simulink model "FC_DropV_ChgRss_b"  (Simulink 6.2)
settings: Solver=ode4  SolverMode=SingleTasking  StartTime=0.0  StopTime=1  FixedStep=1e-5  MaxStep=1e-4  RelTol=1e-3

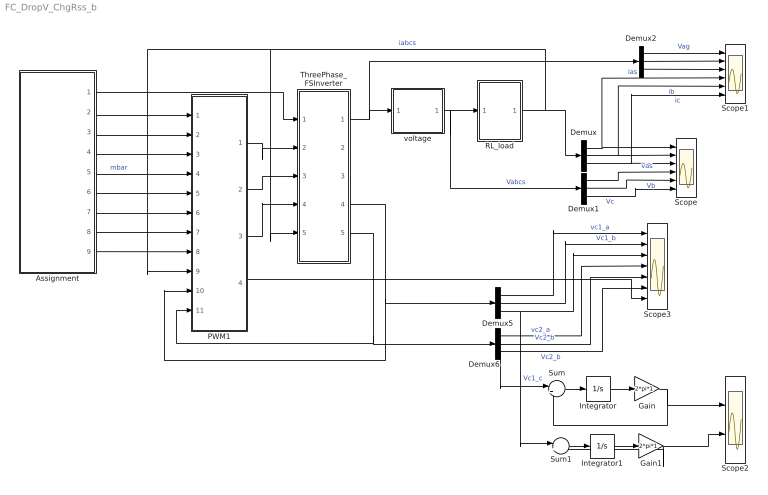
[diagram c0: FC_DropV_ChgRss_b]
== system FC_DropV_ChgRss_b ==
  Assignment : Subsystem  mask{V1Ratio=1, V2Ratio=2, V3Ratio=4, Vdc=50, fe=60, mbar=1.14}
      mask init:
      | Vc1 = Vdc*V1Ratio/V3Ratio;
      | Vc2 = Vdc*V2Ratio/V3Ratio;
  Demux{,1..2,5..6} (5 alike) : Demux  Outputs=3
  Gain : Gain  Gain=2*pi*1
  Gain1 : Gain  Gain=2*pi*1
  Integrator : Integrator
  Integrator1 : Integrator
  PWM1 : Subsystem  AncestorBlock=IMLibrary/PWM1  mask{JustVal=Left Justified, fsw=5e3, F3ndH=on}
      mask prompts: JustVal "Justification"; F3ndH "with the 3nd harmonic injection"
  RL_load : Subsystem  AncestorBlock=IMLibrary/RL_load  mask{Imp=5.37, pf=0.8}
      mask prompts: Imp "Impedance  magnitude"
      mask init:
      | R = pf*Imp;
      | X = sqrt(Imp^2-R^2);
      | L = X/(2*pi*60)
  Scope : Scope  NumInputPorts=6
  Scope1 : Scope  NumInputPorts=6
  Scope2 : Scope  NumInputPorts=2
  Scope3 : Scope  NumInputPorts=7
  Sum : Sum  Inputs=|+-
  Sum1 : Sum  Inputs=|+-
  ThreePhase_FSInverter : Subsystem  AncestorBlock=IMLibrary/ThreePhase_FSInverter  mask{C1=3300e-6, C2=3300e-6, Vc1_a=12.5, Vc2_a=25, Vc1_b=12.5, Vc2_b=25, Vc1_c=12.5, Vc2_c=25}
      mask prompts: Vc1_a "Vc1_a(capacitors initial values)"; Vc2_a "Vc2_a(capacitors initial values)"
  voltage : Subsystem  AncestorBlock=IMLibrary/voltage
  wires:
  Assignment/2(t) -> PWM1/1(t)
  Assignment/4(NLevel) -> PWM1/3(NLevel)
  Assignment/5(mbar) -> PWM1/4(mbar)  "mbar"
  Assignment/6(Vc1_com) -> PWM1/5(V1_com)
  Assignment/7(Vc2_com) -> PWM1/6(V2_com)
  Assignment/8(RSSTable) -> PWM1/7(RSSTable)
  Assignment/9(RSSTable1) -> PWM1/8(RSSTable1)
  Assignment/1(Vdc) -> ThreePhase_FSInverter/1(Vdc)
  ThreePhase_FSInverter/5(Vc2) -> Demux6/1, PWM1/11(V2)
  ThreePhase_FSInverter/4(Vc1) -> Demux5/1, PWM1/10(V1)
  Assignment/3(Theata_c) -> PWM1/2(Theata_c)
  ThreePhase_FSInverter/1(Vabcg) -> Demux2/1, voltage/1(Vabcg)
  PWM1/1(T1) -> ThreePhase_FSInverter/2(T1)
  PWM1/2(T2) -> ThreePhase_FSInverter/3(T2)
  PWM1/3(T3) -> ThreePhase_FSInverter/4(T3)
  voltage/1(Vabcs) -> Demux1/1, RL_load/1(Vabcs)  "Vabcs"
  RL_load/1(iabcs) -> Demux/1, ThreePhase_FSInverter/5(iabcs), PWM1/9(is)  "iabcs"
  Demux/1 -> Scope/1, Scope1/4  "ias"
  Demux/2 -> Scope/2, Scope1/5  "ib"
  Demux/3 -> Scope/3, Scope1/6  "ic"
  Demux2/1 -> Scope1/1  "Vag"
  Demux2/2 -> Scope1/2
  Demux2/3 -> Scope1/3
  PWM1/4(FdeltVPN) -> Scope3/7
  Demux5/3 -> Scope3/3, Sum1/1  "Vc1_c"
  Demux6/3 -> Scope3/6, Sum/1  "Vc2_b"
  Demux5/1 -> Scope3/1  "vc1_a"
  Demux5/2 -> Scope3/2  "Vc1_b"
  Demux6/1 -> Scope3/4  "vc2_a"
  Demux6/2 -> Scope3/5  "Vc2_b"
  Sum/1 -> Integrator/1
  Integrator/1 -> Gain/1
  Gain/1 -> Sum/2, Scope2/1
  Sum1/1 -> Integrator1/1
  Integrator1/1 -> Gain1/1
  Gain1/1 -> Sum1/2, Scope2/2
  Demux1/1 -> Scope/4  "vas"
  Demux1/2 -> Scope/5  "Vb"
  Demux1/3 -> Scope/6  "Vc"

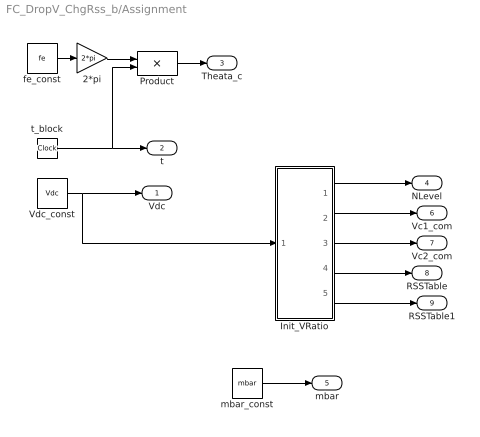
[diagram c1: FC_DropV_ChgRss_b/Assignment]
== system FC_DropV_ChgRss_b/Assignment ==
  2*pi : Gain  Gain=2*pi
  Init_VRatio : Subsystem  AncestorBlock=IMLibrary/Init_VRatio  mask{V1Ratio=V1Ratio, V2Ratio=V2Ratio, V3Ratio=V3Ratio}
  Product : Product
  Vdc_const : Constant  Value=Vdc
  fe_const : Constant  Value=fe
  mbar_const : Constant  Value=mbar
  t_block : Clock
  Vdc : Outport
  t : Outport  Port=2
  Theata_c : Outport  Port=3
  NLevel : Outport  Port=4
  mbar : Outport  Port=5
  Vc1_com : Outport  Port=6
  Vc2_com : Outport  Port=7
  RSSTable : Outport  Port=8
  RSSTable1 : Outport  Port=9
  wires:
  t_block/1 -> t/1, Product/2
  Vdc_const/1 -> Vdc/1, Init_VRatio/1(Vdc)
  Init_VRatio/5(RSSTable1) -> RSSTable1/1
  mbar_const/1 -> mbar/1
  Product/1 -> Theata_c/1
  Init_VRatio/4(RSSTable) -> RSSTable/1
  Init_VRatio/3(Vc2_c) -> Vc2_com/1
  Init_VRatio/2(Vc1_c) -> Vc1_com/1
  Init_VRatio/1(NLevel) -> NLevel/1
  fe_const/1 -> 2*pi/1
  2*pi/1 -> Product/1

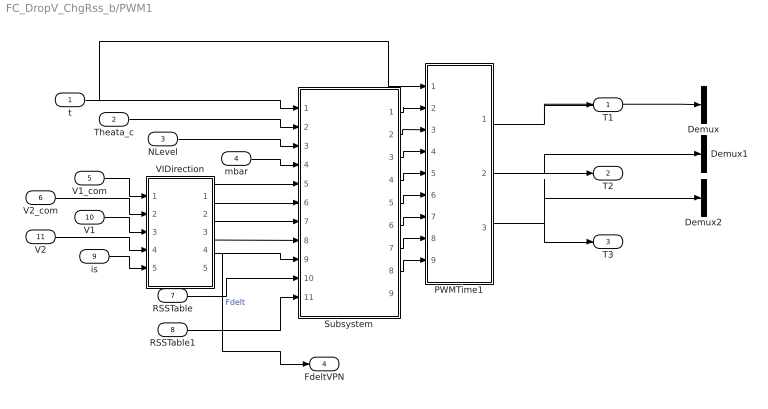
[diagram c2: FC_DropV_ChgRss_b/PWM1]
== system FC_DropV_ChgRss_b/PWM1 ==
  t : Inport  Port=1  LatchInput=off
  Theata_c : Inport  Port=2  LatchInput=off
  NLevel : Inport  Port=3  LatchInput=off
  mbar : Inport  Port=4  LatchInput=off
  V1_com : Inport  Port=5  LatchInput=off
  V2_com : Inport  Port=6  LatchInput=off
  RSSTable : Inport  Port=7  LatchInput=off
  RSSTable1 : Inport  Port=8  LatchInput=off
  is : Inport  Port=9  LatchInput=off
  V1 : Inport  Port=10  LatchInput=off
  V2 : Inport  Port=11  LatchInput=off
  Demux : Demux  Outputs=3
  Demux1 : Demux  Outputs=3
  Demux2 : Demux  Outputs=3
  PWMTime1 : Subsystem
  Subsystem : Subsystem
  VIDirection : Subsystem
  T1 : Outport
  T2 : Outport  Port=2
  T3 : Outport  Port=3
  FdeltVPN : Outport  Port=4
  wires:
  RSSTable1/1 -> Subsystem/11(RSSTable1)
  RSSTable/1 -> Subsystem/10(RSSTable)
  mbar/1 -> Subsystem/4(mbar)
  Theata_c/1 -> Subsystem/2(theta)
  VIDirection/1(FV1) -> Subsystem/5(Fv1)
  VIDirection/2(FV2) -> Subsystem/6(Fv2)
  VIDirection/3(Fis) -> Subsystem/7(Fis)
  V1_com/1 -> VIDirection/1(V1_c)
  V2_com/1 -> VIDirection/2(V2_c)
  is/1 -> VIDirection/5(is)
  VIDirection/4(FDeltVP) -> Subsystem/8(Fdeltp)
  V1/1 -> VIDirection/3(V1)
  V2/1 -> VIDirection/4(V2)
  t/1 -> PWMTime1/1(t), Subsystem/1(t)
  NLevel/1 -> Subsystem/3(NLevel)
  PWMTime1/1(T1) -> T1/1, Demux/1
  PWMTime1/2(T2) -> T2/1, Demux1/1
  PWMTime1/3(T3) -> T3/1, Demux2/1
  VIDirection/5(FDeltVPN) -> FdeltVPN/1, Subsystem/9(FdeltVPN)  "Fdelt"
  Subsystem/1(Row_a) -> PWMTime1/2(Row_a)
  Subsystem/2(Row_b) -> PWMTime1/3(Row_b)
  Subsystem/3(Row_c) -> PWMTime1/4(Row_c)
  Subsystem/4(t1) -> PWMTime1/5(time1)
  Subsystem/5(t2) -> PWMTime1/6(time2)
  Subsystem/6(t3) -> PWMTime1/7(time3)
  Subsystem/7(TPos) -> PWMTime1/8(Tpos)
  Subsystem/8(AlterIndex) -> PWMTime1/9(AlterIndex)

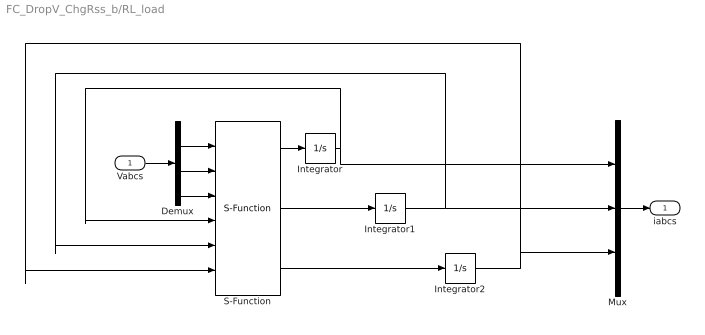
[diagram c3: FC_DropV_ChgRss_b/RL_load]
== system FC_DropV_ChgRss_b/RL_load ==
  Vabcs : Inport  Port=1  LatchInput=off
  Demux : Demux  Outputs=3
  Integrator : Integrator
  Integrator1 : Integrator
  Integrator2 : Integrator
  Mux : Mux  Inputs=3
  S-Function : S-Function  FunctionName=RL_load  Parameters=R,L
  iabcs : Outport
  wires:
  Mux/1 -> iabcs/1
  Vabcs/1 -> Demux/1
  Demux/3 -> S-Function/3
  Demux/2 -> S-Function/2
  Demux/1 -> S-Function/1
  Integrator2/1 -> Mux/3, S-Function/6
  S-Function/3 -> Integrator2/1
  Integrator1/1 -> Mux/2, S-Function/5
  S-Function/2 -> Integrator1/1
  Integrator/1 -> Mux/1, S-Function/4
  S-Function/1 -> Integrator/1

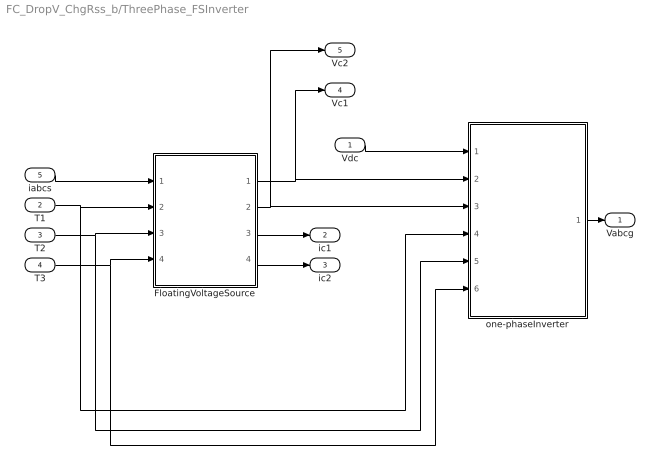
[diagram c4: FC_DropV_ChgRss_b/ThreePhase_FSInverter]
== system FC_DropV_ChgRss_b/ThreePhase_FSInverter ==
  Vdc : Inport  Port=1  LatchInput=off
  T1 : Inport  Port=2  LatchInput=off
  T2 : Inport  Port=3  LatchInput=off
  T3 : Inport  Port=4  LatchInput=off
  iabcs : Inport  Port=5  LatchInput=off
  FloatingVoltageSource : Subsystem  mask{C1=C1, C2=C2, Vc1_a=Vc1_a, Vc2_a=Vc2_a, Vc1_b=Vc1_b, Vc2_b=Vc2_b, Vc1_c=Vc1_c, Vc2_c=Vc2_c}
      mask prompts: Vc1_a "Vc1_a(capacitors initial values)"; Vc2_a "Vc2_a(capacitors initial values)"
  one-phaseInverter : Subsystem
  Vabcg : Outport
  ic1 : Outport  Port=2
  ic2 : Outport  Port=3
  Vc1 : Outport  Port=4
  Vc2 : Outport  Port=5
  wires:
  one-phaseInverter/1(Vabcg) -> Vabcg/1
  FloatingVoltageSource/2(Vc2_abc) -> Vc2/1, one-phaseInverter/3(Vc2)
  FloatingVoltageSource/1(Vc1_abc) -> Vc1/1, one-phaseInverter/2(Vc1)
  FloatingVoltageSource/4(ic2) -> ic2/1
  FloatingVoltageSource/3(ic1) -> ic1/1
  iabcs/1 -> FloatingVoltageSource/1(iabcs)
  Vdc/1 -> one-phaseInverter/1(Vdc)
  T3/1 -> one-phaseInverter/6(T3), FloatingVoltageSource/4(T3)
  T2/1 -> one-phaseInverter/5(T2), FloatingVoltageSource/3(T2)
  T1/1 -> one-phaseInverter/4(T1), FloatingVoltageSource/2(T1)

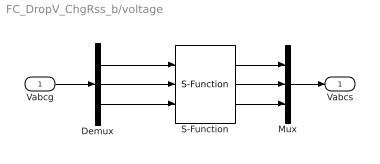
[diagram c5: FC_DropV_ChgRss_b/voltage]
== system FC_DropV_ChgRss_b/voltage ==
  Vabcg : Inport  Port=1  LatchInput=off
  Demux : Demux  Outputs=3
  Mux : Mux  Inputs=3
  S-Function : S-Function  FunctionName=voltage
  Vabcs : Outport
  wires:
  Vabcg/1 -> Demux/1
  Demux/2 -> S-Function/2
  Mux/1 -> Vabcs/1
  S-Function/3 -> Mux/3
  S-Function/2 -> Mux/2
  Demux/3 -> S-Function/3
  S-Function/1 -> Mux/1
  Demux/1 -> S-Function/1

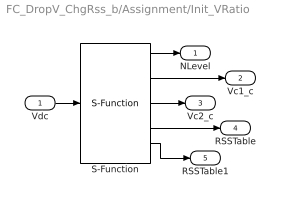
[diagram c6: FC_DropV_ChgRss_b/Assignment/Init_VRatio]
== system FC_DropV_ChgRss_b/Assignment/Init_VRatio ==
  Vdc : Inport  Port=1  LatchInput=off
  S-Function : S-Function  FunctionName=Init_VRatio_ChgRss_b  Parameters=V1Ratio,V2Ratio,V3Ratio  mask{V1Ratio=V1Ratio, V2Ratio=V2Ratio, V3Ratio=V3Ratio}
  NLevel : Outport
  Vc1_c : Outport  Port=2
  Vc2_c : Outport  Port=3
  RSSTable : Outport  Port=4
  RSSTable1 : Outport  Port=5
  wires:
  S-Function/5 -> RSSTable1/1
  S-Function/4 -> RSSTable/1
  S-Function/3 -> Vc2_c/1
  S-Function/2 -> Vc1_c/1
  Vdc/1 -> S-Function/1
  S-Function/1 -> NLevel/1

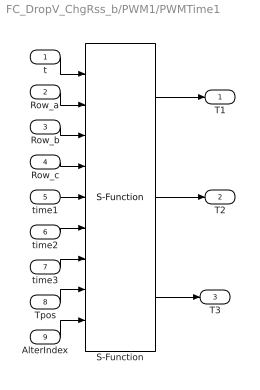
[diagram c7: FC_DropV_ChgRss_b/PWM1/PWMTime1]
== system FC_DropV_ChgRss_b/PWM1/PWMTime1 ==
  t : Inport  Port=1  LatchInput=off
  Row_a : Inport  Port=2  LatchInput=off
  Row_b : Inport  Port=3  LatchInput=off
  Row_c : Inport  Port=4  LatchInput=off
  time1 : Inport  Port=5  LatchInput=off
  time2 : Inport  Port=6  LatchInput=off
  time3 : Inport  Port=7  LatchInput=off
  Tpos : Inport  Port=8  LatchInput=off
  AlterIndex : Inport  Port=9  LatchInput=off
  S-Function : S-Function  FunctionName=PWMTime1  Parameters=JustVal,fsw
  T1 : Outport
  T2 : Outport  Port=2
  T3 : Outport  Port=3
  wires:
  S-Function/3 -> T3/1
  S-Function/2 -> T2/1
  AlterIndex/1 -> S-Function/9
  Tpos/1 -> S-Function/8
  time3/1 -> S-Function/7
  time2/1 -> S-Function/6
  time1/1 -> S-Function/5
  Row_c/1 -> S-Function/4
  Row_b/1 -> S-Function/3
  Row_a/1 -> S-Function/2
  S-Function/1 -> T1/1
  t/1 -> S-Function/1

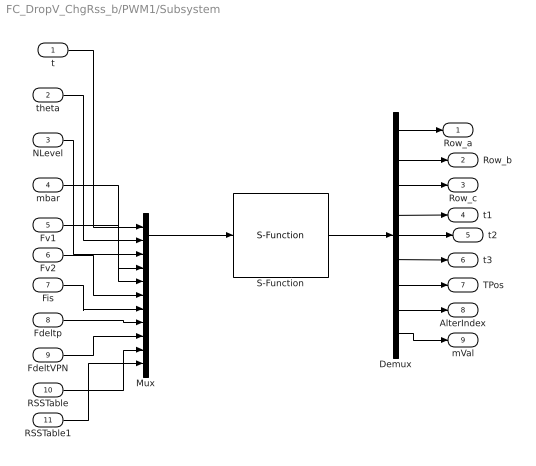
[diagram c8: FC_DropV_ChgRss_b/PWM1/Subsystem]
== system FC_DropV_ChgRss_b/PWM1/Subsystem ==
  t : Inport  Port=1  LatchInput=off
  theta : Inport  Port=2  LatchInput=off
  NLevel : Inport  Port=3  LatchInput=off
  mbar : Inport  Port=4  LatchInput=off
  Fv1 : Inport  Port=5  LatchInput=off
  Fv2 : Inport  Port=6  LatchInput=off
  Fis : Inport  Port=7  LatchInput=off
  Fdeltp : Inport  Port=8  LatchInput=off
  FdeltVPN : Inport  Port=9  LatchInput=off
  RSSTable : Inport  Port=10  LatchInput=off
  RSSTable1 : Inport  Port=11  LatchInput=off
  Demux : Demux  Outputs=[4,4,4,1,1,1,1,1,1]
  Mux : Mux  Inputs=[1,1,1,1,3,3,3,3,1,128,98304]
  S-Function : S-Function  FunctionName=PWMControl_bM  Parameters=JustVal,fsw,F3ndH
  Row_a : Outport
  Row_b : Outport  Port=2
  Row_c : Outport  Port=3
  t1 : Outport  Port=4
  t2 : Outport  Port=5
  t3 : Outport  Port=6
  TPos : Outport  Port=7
  AlterIndex : Outport  Port=8
  mVal : Outport  Port=9
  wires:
  Mux/1 -> S-Function/1
  S-Function/1 -> Demux/1
  Demux/1 -> Row_a/1
  Demux/2 -> Row_b/1
  Demux/3 -> Row_c/1
  Demux/4 -> t1/1
  Demux/5 -> t2/1
  Demux/6 -> t3/1
  Demux/7 -> TPos/1
  Demux/8 -> AlterIndex/1
  Demux/9 -> mVal/1
  t/1 -> Mux/1
  theta/1 -> Mux/2
  NLevel/1 -> Mux/3
  mbar/1 -> Mux/4
  Fv1/1 -> Mux/5
  Fv2/1 -> Mux/6
  Fis/1 -> Mux/7
  Fdeltp/1 -> Mux/8
  FdeltVPN/1 -> Mux/9
  RSSTable/1 -> Mux/10
  RSSTable1/1 -> Mux/11

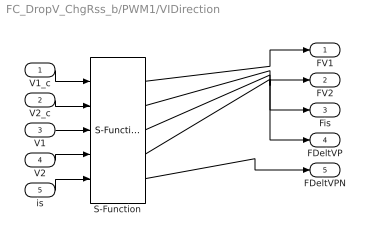
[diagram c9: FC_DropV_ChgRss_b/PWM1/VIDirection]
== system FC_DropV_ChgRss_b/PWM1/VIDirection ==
  V1_c : Inport  Port=1  LatchInput=off
  V2_c : Inport  Port=2  LatchInput=off
  V1 : Inport  Port=3  LatchInput=off
  V2 : Inport  Port=4  LatchInput=off
  is : Inport  Port=5  LatchInput=off
  S-Function : S-Function  FunctionName=VIDirection_drop
  FV1 : Outport
  FV2 : Outport  Port=2
  Fis : Outport  Port=3
  FDeltVP : Outport  Port=4
  FDeltVPN : Outport  Port=5
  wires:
  V1_c/1 -> S-Function/1
  S-Function/1 -> FV1/1
  V2_c/1 -> S-Function/2
  V1/1 -> S-Function/3
  S-Function/2 -> FV2/1
  V2/1 -> S-Function/4
  S-Function/3 -> Fis/1
  is/1 -> S-Function/5
  S-Function/4 -> FDeltVP/1
  S-Function/5 -> FDeltVPN/1

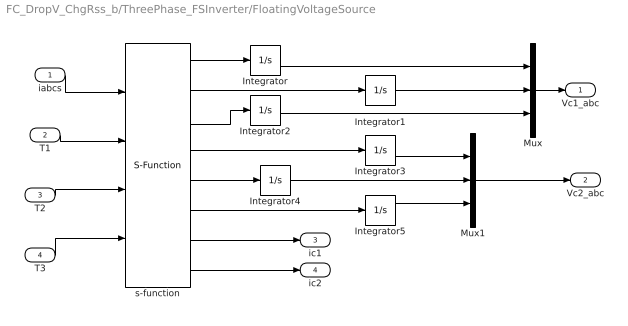
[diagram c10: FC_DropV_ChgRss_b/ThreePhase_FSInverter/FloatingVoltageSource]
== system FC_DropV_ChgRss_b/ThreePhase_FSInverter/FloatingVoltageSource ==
  iabcs : Inport  Port=1  LatchInput=off
  T1 : Inport  Port=2  LatchInput=off
  T2 : Inport  Port=3  LatchInput=off
  T3 : Inport  Port=4  LatchInput=off
  Integrator : Integrator  InitialCondition=Vc1_a
  Integrator1 : Integrator  InitialCondition=Vc1_b
  Integrator2 : Integrator  InitialCondition=Vc1_c
  Integrator3 : Integrator  InitialCondition=Vc2_a
  Integrator4 : Integrator  InitialCondition=Vc2_b
  Integrator5 : Integrator  InitialCondition=Vc2_c
  Mux : Mux  Inputs=3
  Mux1 : Mux  Inputs=3
  s-function : S-Function  FunctionName=FloatingVSrc  Parameters=C1,C2  mask{C1=C1, C2=C2}
  Vc1_abc : Outport
  Vc2_abc : Outport  Port=2
  ic1 : Outport  Port=3
  ic2 : Outport  Port=4
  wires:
  Mux/1 -> Vc1_abc/1
  Mux1/1 -> Vc2_abc/1
  Integrator4/1 -> Mux1/2
  s-function/8 -> ic2/1
  s-function/7 -> ic1/1
  s-function/6 -> Integrator5/1
  s-function/5 -> Integrator4/1
  Integrator5/1 -> Mux1/3
  Integrator3/1 -> Mux1/1
  s-function/4 -> Integrator3/1
  Integrator2/1 -> Mux/3
  s-function/3 -> Integrator2/1
  T2/1 -> s-function/3
  T1/1 -> s-function/2
  T3/1 -> s-function/4
  iabcs/1 -> s-function/1
  Integrator1/1 -> Mux/2
  s-function/2 -> Integrator1/1
  Integrator/1 -> Mux/1
  s-function/1 -> Integrator/1

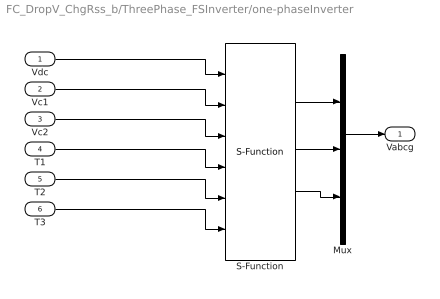
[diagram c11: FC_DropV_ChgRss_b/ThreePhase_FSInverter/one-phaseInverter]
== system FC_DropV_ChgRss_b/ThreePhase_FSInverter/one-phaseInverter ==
  Vdc : Inport  Port=1  LatchInput=off
  Vc1 : Inport  Port=2  LatchInput=off
  Vc2 : Inport  Port=3  LatchInput=off
  T1 : Inport  Port=4  LatchInput=off
  T2 : Inport  Port=5  LatchInput=off
  T3 : Inport  Port=6  LatchInput=off
  Mux : Mux  Inputs=3
  S-Function : S-Function  FunctionName=Inverter
  Vabcg : Outport
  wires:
  Mux/1 -> Vabcg/1
  S-Function/3 -> Mux/3
  S-Function/2 -> Mux/2
  T3/1 -> S-Function/6
  T2/1 -> S-Function/5
  T1/1 -> S-Function/4
  Vc2/1 -> S-Function/3
  S-Function/1 -> Mux/1
  Vc1/1 -> S-Function/2
  Vdc/1 -> S-Function/1
